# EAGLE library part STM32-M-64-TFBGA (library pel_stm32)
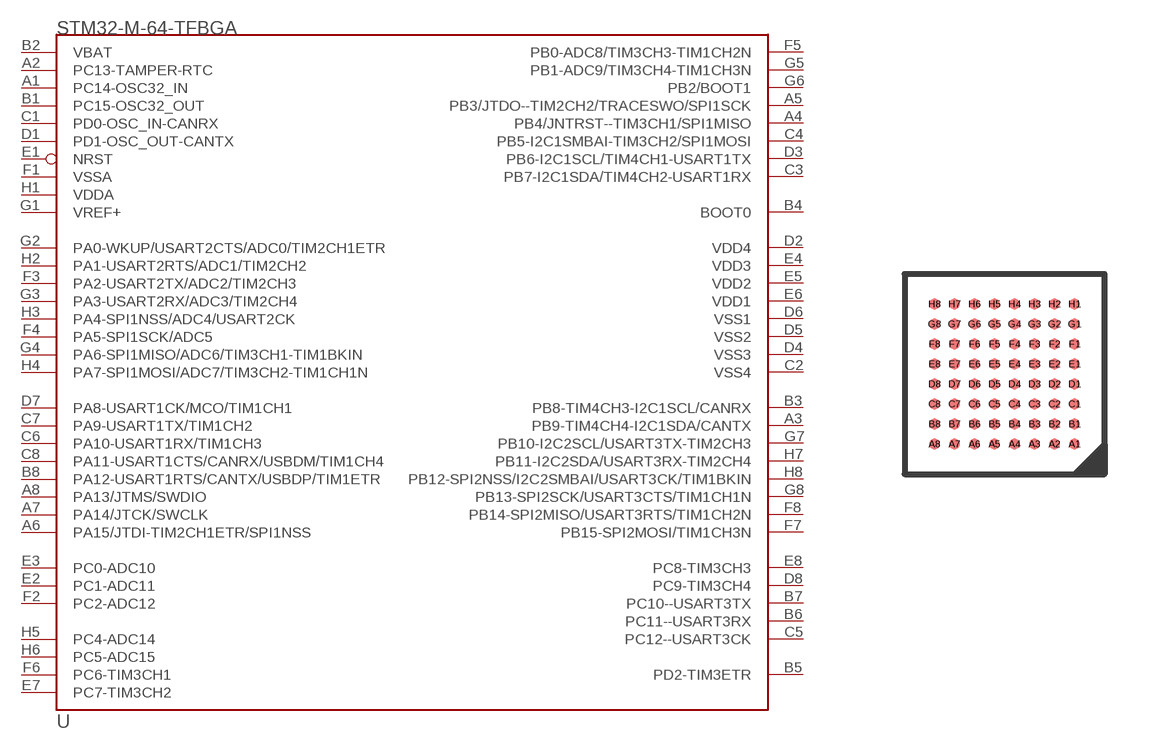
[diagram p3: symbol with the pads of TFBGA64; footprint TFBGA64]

Designator prefix U

## STM32-M-64-TFBGA  [TFBGA64]
A1  PC14-OSC32_IN
A2  PC13-TAMPER-RTC
A3  PB9-TIM4CH4-I2C1SDA/CANTX
A4  PB4/JNTRST--TIM3CH1/SPI1MISO
A5  PB3/JTDO--TIM2CH2/TRACESWO/SPI1SCK
A6  PA15/JTDI-TIM2CH1ETR/SPI1NSS
A7  PA14/JTCK/SWCLK
A8  PA13/JTMS/SWDIO
B1  PC15-OSC32_OUT
B2  VBAT  sup
B3  PB8-TIM4CH3-I2C1SCL/CANRX
B4  BOOT0  in
B5  PD2-TIM3ETR
B6  PC11--USART3RX
B7  PC10--USART3TX
B8  PA12-USART1RTS/CANTX/USBDP/TIM1ETR
C1  PD0-OSC_IN-CANRX  in
C2  VSS4
C3  PB7-I2C1SDA/TIM4CH2-USART1RX
C4  PB5-I2C1SMBAI-TIM3CH2/SPI1MOSI
C5  PC12--USART3CK
C6  PA10-USART1RX/TIM1CH3
C7  PA9-USART1TX/TIM1CH2
C8  PA11-USART1CTS/CANRX/USBDM/TIM1CH4
D1  PD1-OSC_OUT-CANTX  out
D2  VDD4
D3  PB6-I2C1SCL/TIM4CH1-USART1TX
D4  VSS3  sup
D5  VSS2  sup
D6  VSS1  sup
D7  PA8-USART1CK/MCO/TIM1CH1
D8  PC9-TIM3CH4
E1  NRST
E2  PC1-ADC11
E3  PC0-ADC10
E4  VDD3  sup
E5  VDD2  sup
E6  VDD1  sup
E7  PC7-TIM3CH2
E8  PC8-TIM3CH3
F1  VSSA  sup
F2  PC2-ADC12
F3  PA2-USART2TX/ADC2/TIM2CH3
F4  PA5-SPI1SCK/ADC5
F5  PB0-ADC8/TIM3CH3-TIM1CH2N
F6  PC6-TIM3CH1
F7  PB15-SPI2MOSI/TIM1CH3N
F8  PB14-SPI2MISO/USART3RTS/TIM1CH2N
G1  VREF+
G2  PA0-WKUP/USART2CTS/ADC0/TIM2CH1ETR
G3  PA3-USART2RX/ADC3/TIM2CH4
G4  PA6-SPI1MISO/ADC6/TIM3CH1-TIM1BKIN
G5  PB1-ADC9/TIM3CH4-TIM1CH3N
G6  PB2/BOOT1
G7  PB10-I2C2SCL/USART3TX-TIM2CH3
G8  PB13-SPI2SCK/USART3CTS/TIM1CH1N
H1  VDDA  sup
H2  PA1-USART2RTS/ADC1/TIM2CH2
H3  PA4-SPI1NSS/ADC4/USART2CK
H4  PA7-SPI1MOSI/ADC7/TIM3CH2-TIM1CH1N
H5  PC4-ADC14
H6  PC5-ADC15
H7  PB11-I2C2SDA/USART3RX-TIM2CH4
H8  PB12-SPI2NSS/I2C2SMBAI/USART3CK/TIM1BKIN

## Footprint TFBGA64 (pad centres in mm)
smd 0.27 x 0.27: A1 1.75,-1.75; A2 1.25,-1.75; A3 0.75,-1.75; A4 0.25,-1.75; A5 -0.25,-1.75; A6 -0.75,-1.75; A7 -1.25,-1.75; A8 -1.75,-1.75; B1 1.75,-1.25; B2 1.25,-1.25; B3 0.75,-1.25; B4 0.25,-1.25; B5 -0.25,-1.25; B6 -0.75,-1.25; B7 -1.25,-1.25; B8 -1.75,-1.25; C1 1.75,-0.75; C2 1.25,-0.75; C3 0.75,-0.75; C4 0.25,-0.75; C5 -0.25,-0.75; C6 -0.75,-0.75; C7 -1.25,-0.75; C8 -1.75,-0.75; D1 1.75,-0.25; D2 1.25,-0.25; D3 0.75,-0.25; D4 0.25,-0.25; D5 -0.25,-0.25; D6 -0.75,-0.25; D7 -1.25,-0.25; D8 -1.75,-0.25; E1 1.75,0.25; E2 1.25,0.25; E3 0.75,0.25; E4 0.25,0.25; E5 -0.25,0.25; E6 -0.75,0.25; E7 -1.25,0.25; E8 -1.75,0.25; F1 1.75,0.75; F2 1.25,0.75; F3 0.75,0.75; F4 0.25,0.75; F5 -0.25,0.75; F6 -0.75,0.75; F7 -1.25,0.75; F8 -1.75,0.75; G1 1.75,1.25; G2 1.25,1.25; G3 0.75,1.25; G4 0.25,1.25; G5 -0.25,1.25; G6 -0.75,1.25; G7 -1.25,1.25; G8 -1.75,1.25; H1 1.75,1.75; H2 1.25,1.75; H3 0.75,1.75; H4 0.25,1.75; H5 -0.25,1.75; H6 -0.75,1.75; H7 -1.25,1.75; H8 -1.75,1.75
